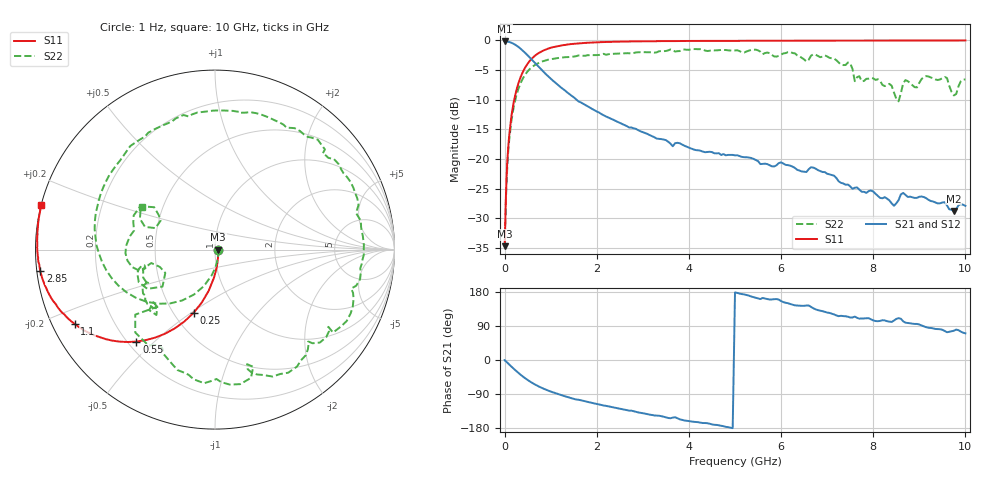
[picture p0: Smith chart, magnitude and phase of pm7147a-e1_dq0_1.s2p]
# GHz S DB R 50
! S-Parameters data
! Freq  dbS11  angS11  dbS21  angS21  dbS12  angS12  dbS22  angS22
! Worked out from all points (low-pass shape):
!   279 points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, 1 Hz to 10 GHz, reference 50 ohm
!   highest |S21| = -0.16 dB at 6.31 kHz (marker M1); lowest = -28.8 dB at 9.75 GHz (marker M2)
!   |S21| within 3 dB of the highest: start of sweep to 579 MHz
!   lowest |S11| = -34.7 dB at 6.31 kHz (marker M3), VSWR 1.04, Z = 51.9 - j0.000932 ohm
!   |S11| at or under -10 dB: start of sweep to 209.2 MHz
!   |S22| runs from -34.7 to -1.5 dB; largest |S21 - S12| = 1.1e-11
!   S11 on the Smith chart (normalised r, x): 1 Hz: 1.04, -0.00; 250 MHz: 0.62, -0.51; 550 MHz: 0.23, -0.44; 1.1 GHz: 0.06, -0.25; 2.85 GHz: 0.01, -0.06; 10 GHz: 0.00, +0.13
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1e-09  -34.73 -0.0  -0.16 0.0  -0.16 0.0  -34.73 -0.0
6.3096e-06  -34.73 -0.0  -0.16 -0.0  -0.16 -0.0  -34.73 -0.0
0.03981072  -23.64 -77.0  -0.18 -4.8  -0.18 -4.8  -24.33 -77.9
0.07943282  -17.95 -88.8  -0.23 -9.5  -0.23 -9.5  -18.68 -92.6
0.25  -8.58 -108.8  -0.84 -28.9  -0.84 -28.9  -9.45 -122.8
0.55  -3.43 -130.5  -2.93 -56.8  -2.93 -56.8  -4.81 -159.7
1.1  -1.06 -152.2  -7.13 -87.4  -7.13 -87.4  -3.05 156.9
1.7  -0.45 -163.0  -10.67 -107.6  -10.67 -107.6  -2.59 124.0
2.85  -0.17 -173.1  -14.93 -136.7  -14.93 -136.7  -2.04 75.7
3.35  -0.13 -175.7  -16.61 -147.1  -16.61 -147.1  -1.84 56.8
4.25  -0.09 -179.5  -18.62 -165.3  -18.62 -165.3  -1.49 19.7
5.05  -0.08 177.8  -19.39 177.0  -19.39 177.0  -1.67 -11.6
5.55  -0.06 176.4  -20.88 160.8  -20.88 160.8  -1.90 -35.1
6.7  -0.05 173.3  -21.46 136.5  -21.46 136.5  -2.35 -79.4
7.5  -0.03 171.4  -24.64 112.1  -24.64 112.1  -3.87 -133.9
7.6  -0.03 171.1  -24.86 114.5  -24.86 114.5  -6.89 -135.3
8.35  -0.02 169.3  -27.00 101.3  -27.00 101.3  -7.34 -158.7
8.55  -0.02 168.9  -26.97 110.4  -26.97 110.4  -10.29 -154.9
8.7  -0.02 168.6  -26.07 98.4  -26.07 98.4  -6.71 -156.8
9.2  -0.02 167.5  -26.91 85.0  -26.91 85.0  -6.09 177.7
9.75  -0.01 166.3  -28.81 77.2  -28.81 77.2  -9.29 152.0
10  -0.02 165.7  -27.93 70.4  -27.93 70.4  -6.59 149.7
